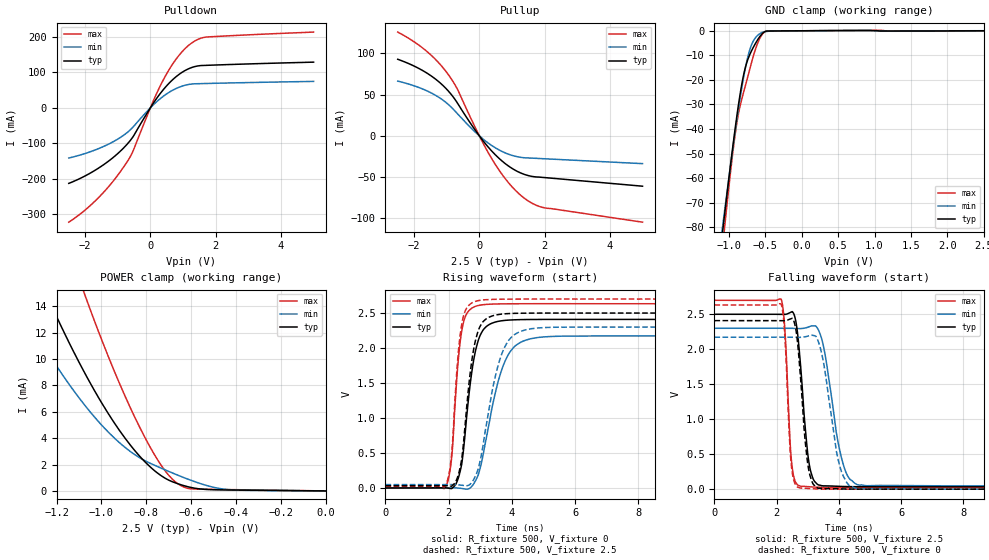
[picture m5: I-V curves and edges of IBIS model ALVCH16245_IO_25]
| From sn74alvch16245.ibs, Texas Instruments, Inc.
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[Model]   ALVCH16245_IO_25
Model_type  I/O
Vinl=0.7
Vinh=1.7
Enable   Active-Low
Vref =   0
Rref =   500
Cref =   30p
Vmeas =   1.25
| variable   typ   min   max
C_comp   8.26pF   7.17pF   9.31pF
| C_pullup   9.45pF   7.80pF   10.46pF
| C_pulldown   12.07pF   9.62pF   15.22pF
| C_tri-state   8.26pF   7.17pF   9.31pF
[Temperature Range]   40   100   -40
| Ambient temperature   25   85   -40
[Voltage range]   2.5   2.3   2.7
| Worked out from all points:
|   slope of the pulldown table from 0 to 0.375 V, typ, clamps not added: 7.66 ohm
|   slope of the pullup table from 0 to 0.375 V, typ, clamps not added: 20.6 ohm
|   GND clamp passes 1 mA (typ) near -0.54 V on its own axis
|   POWER clamp passes 1 mA (typ) near -0.72 V on its own axis
|   rising waveform, R_fixture 500, V_fixture 0: 20-80 % time 380ps typ, 645ps min, 257ps max; typ from 0 V to 2.41 V
|   falling waveform, R_fixture 500, V_fixture 2.5: 20-80 % time 272ps typ, 472ps min, 168ps max; typ from 2.5 V to 0.034 V
|   rising waveform, R_fixture 500, V_fixture 2.5: 20-80 % time 358ps typ, 585ps min, 250ps max; typ from 0.034 V to 2.5 V
|   falling waveform, R_fixture 500, V_fixture 0: 20-80 % time 259ps typ, 437ps min, 164ps max; typ from 2.41 V to 0 V
[GND Clamp]
| ALVCH16245_IO_25
|   Voltage   I(typ)   I(min)   I(max)
-2.5V     -485mA     -444.7mA   -547.1mA
-1.085V   -81.07mA   -78.95mA   -87.25mA
-1.07V    -77.22mA   -75.45mA   -82.89mA
-1.05V    -72.13mA   -70.82mA   -77.14mA
-915mV    -39.69mA   -41mA      -42.06mA
-870mV    -30.15mA   -31.86mA   -33.77mA
-810mV    -19.51mA   -20.77mA   -26.19mA
-745mV    -12.02mA   -11.07mA   -19.05mA
-695mV    -8.455mA   -6.064mA   -13.44mA
-555mV    -1.559mA   -802.7uA   -1.963mA
-420mV    -88.65uA   -111.7uA   -126.8uA
2.5V      87.97pA    20.8uA     -42.68uA
[POWER Clamp]
| ALVCH16245_IO_25
|   Voltage   I(typ)   I(min)   I(max)
-2.5V     78.71mA    58.49mA    109mA
-1.385V   20.48mA    14.69mA    31.36mA
-1.24V    14.7mA     10.52mA    23.24mA
-1.08V    9.114mA    6.62mA     15.15mA
-1.065V   8.641mA    6.299mA    14.44mA
-945mV    5.218mA    4.051mA    9.173mA
-855mV    3.133mA    2.791mA    5.716mA
-755mV    1.42mA     1.885mA    2.505mA
-670mV    609.2uA    1.265mA    681.5uA
-605mV    277uA      830.7uA    166.5uA
-445mV    73.42uA    118.1uA    104.1uA
-31.15fV  87.97pA    327.7pA    50.89pA
[Pulldown]
| ALVCH16245_IO_25
|   Voltage   I(typ)   I(min)   I(max)
-2.5V     -213.5mA   -141.7mA   -323.1mA
-1.595V   -170.7mA   -115.5mA   -254.3mA
-1.18V    -143.3mA   -97.74mA   -211.7mA
-805mV    -111.9mA   -76.42mA   -165.1mA
-545mV    -83.42mA   -55.66mA   -124.8mA
70mV      10.13mA    6.566mA    15.4mA
425mV     54.54mA    34.7mA     83.99mA
820mV     90.47mA    55.98mA    141.7mA
1.215V    112.2mA    66.71mA    179.9mA
1.465V    118.6mA    68.28mA    193.9mA
1.715V    120.1mA    68.86mA    200.1mA
5V        129.2mA    74.77mA    214.1mA
[Pullup]
| ALVCH16245_IO_25
|   Voltage   I(typ)   I(min)   I(max)
-2.5V     92.96mA    66.45mA    126mA
-1.66V    77.48mA    55.56mA    104.2mA
-1.315V   68.02mA    48.56mA    91.64mA
-1.01V    56.98mA    40.11mA    77.55mA
-685mV    40.61mA    27.47mA    57.59mA
15mV      -812.9uA   -531.7uA   -1.2mA
425mV     -20.36mA   -12.93mA   -30.68mA
890mV     -36.57mA   -22.24mA   -56.75mA
1.36V     -46.54mA   -26.55mA   -75.17mA
1.67V     -49.6mA    -27.19mA   -82.95mA
1.985V    -50.63mA   -27.82mA   -87.32mA
5V        -61.14mA   -33.76mA   -104.8mA
[Ramp]
| ALVCH16245_IO_25
| variable   typ   min   max
dV/dt_r   1.45/3.97E-10   1.31/6.76E-10   1.59/2.64E-10
dV/dt_f   1.50/2.82E-10   1.37/5.12E-10   1.62/1.77E-10
R_load = 500
[Rising Waveform]
| ALVCH16245_IO_25
R_fixture =   500
C_fixture =   0
L_fixture =   0
V_fixture =   0
V_fixture_min = 0
V_fixture_max = 0
|   Time   V(typ)   V(min)   V(max)
0s        360.6pV    1.412nV    255.5pV
1.91ns    1.033mV    581.2uV    22.05mV
2.1ns     -6.603mV   2.002mV    461.6mV
2.285ns   116.9mV    -1.111mV   1.734V
2.44ns    434.8mV    -9.263mV   2.31V
2.76ns    1.746V     39.78mV    2.578V
3.07ns    2.245V     430.9mV    2.619V
3.84ns    2.398V     1.867V     2.632V
4.99ns    2.409V     2.159V     2.634V
50ns      2.409V     2.172V     2.633V
[Falling Waveform]
| ALVCH16245_IO_25
R_fixture =   500
C_fixture =   0
L_fixture =   0
V_fixture =   2.5
V_fixture_min = 2.3
V_fixture_max = 2.7
|   Time   V(typ)   V(min)   V(max)
0s        2.5V       2.3V       2.7V
2.15ns    2.499V     2.3V       2.713V
2.275ns   2.499V     2.3V       2.211V
2.485ns   2.535V     2.299V     370.1mV
2.785ns   1.683V     2.296V     41.64mV
3.19ns    131.4mV    2.335V     30.77mV
3.505ns   46.92mV    2.045V     26.13mV
4.135ns   38.45mV    364.2mV    24.23mV
4.655ns   34.67mV    57.58mV    23.96mV
50ns      33.66mV    47.56mV    23.96mV
[Rising Waveform]
| ALVCH16245_IO_25
R_fixture =   500
C_fixture =   0
L_fixture =   0
V_fixture =   2.5
V_fixture_min = 2.3
V_fixture_max = 2.7
|   Time   V(typ)   V(min)   V(max)
0s        33.65mV    47.56mV    23.96mV
1.905ns   34.21mV    47.63mV    42.91mV
2.09ns    24.63mV    48.26mV    472.4mV
2.28ns    154.1mV    44.94mV    1.809V
2.435ns   498.6mV    37.76mV    2.393V
2.74ns    1.845V     84.81mV    2.646V
3.05ns    2.354V     513.8mV    2.686V
3.735ns   2.488V     1.978V     2.699V
4.805ns   2.5V       2.286V     2.7V
50ns      2.5V       2.3V       2.7V
[Falling Waveform]
| ALVCH16245_IO_25
R_fixture =   500
C_fixture =   0
L_fixture =   0
V_fixture =   0
V_fixture_min = 0
V_fixture_max = 0
|   Time   V(typ)   V(min)   V(max)
0s        2.409V     2.172V     2.633V
2.15ns    2.408V     2.172V     2.643V
2.265ns   2.409V     2.172V     2.175V
2.475ns   2.438V     2.172V     331.1mV
2.775ns   1.556V     2.17V      15.57mV
3.165ns   79.83mV    2.198V     6.097mV
3.47ns    7.338mV    1.895V     1.878mV
4.045ns   4.354mV    306.5mV    254.2uV
4.61ns    666.4uV    4.89mV     -14.29uV
50ns      244.2nV    449.9nV    121nV
